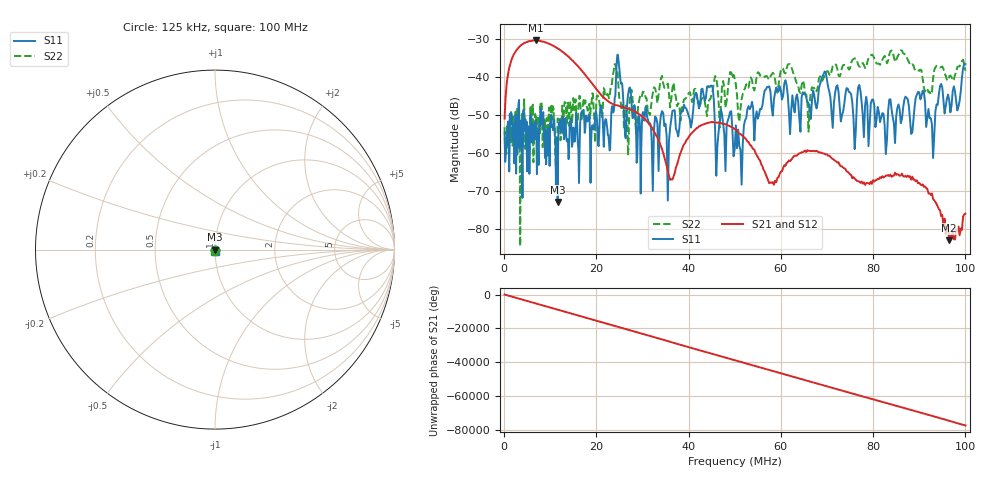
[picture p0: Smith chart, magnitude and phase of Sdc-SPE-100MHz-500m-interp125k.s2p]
!Keysight Technologies PLTS 2019, Build 20190114.1
!FILE: C:\Users\fxb06141\Documents\BUREAU - 2022\IEEE802.3\IEEE802.3dg\Cable modeling\125kHz Interpolation\SPE-100MHz-500m-interp125k.s4p
!$DUT_CFG_DESC: Default 4-Port Configuration
!$NUMBER_PORTS: 4
!$DIFF_PORT_MAP: 1|2P|2|2P|0|UC|0|UC|
!$PORT_MAP: 1|1|<<<<<<|2|2|>>>>>>|3|3|<<<<<<|4|4|>>>>>>|
!Date: Tuesday, March 05, 2024, 10:50:46
!S2P File: Measurements: SDC11,SDC12,SDC21,SDC22:
# MHz S  RI  R 50
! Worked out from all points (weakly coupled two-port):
!   800 points, 125 kHz to 100 MHz, reference 50 ohm
!   highest |S21| = -30.26 dB at 6.875 MHz (marker M1); lowest = -83.0 dB at 96.5 MHz (marker M2)
!   lowest |S11| = -72.9 dB at 11.62 MHz (marker M3), VSWR 1.00, Z = 50 + j0.00189 ohm
!   |S11| at or under -10 dB: start of sweep to end of sweep
!   |S22| runs from -84.6 to -32.9 dB; largest |S21 - S12| = 0
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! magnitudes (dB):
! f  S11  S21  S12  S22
! 125 kHz  -54.6  -50.9  -50.9  -53.2
! 2 MHz  -52.3  -34.2  -34.2  -50.3
! 6.875 MHz  -51.3  -30.3  -30.3  -51.8
! 11.62 MHz  -72.9  -32.3  -32.3  -50.8
! 16.88 MHz  -49.1  -38.3  -38.3  -51.3
! 22.75 MHz  -57.1  -46.5  -46.5  -45.6
! 24.75 MHz  -34.8  -47.5  -47.5  -41.3
! 26.5 MHz  -52.4  -48.1  -48.1  -47.5
! 29.25 MHz  -50.0  -49.7  -49.7  -46.4
! 33.5 MHz  -64.7  -56.7  -56.7  -44.6
! 36.38 MHz  -49.9  -67.0  -67.0  -44.2
! 44.62 MHz  -42.4  -51.9  -51.9  -45.8
! 46.12 MHz  -62.0  -51.9  -51.9  -41.3
! 50.12 MHz  -55.8  -53.7  -53.7  -41.1
! 58 MHz  -47.9  -67.8  -67.8  -39.3
! 66.75 MHz  -46.0  -59.4  -59.4  -42.6
! 69.38 MHz  -38.8  -60.1  -60.1  -39.8
! 75.88 MHz  -55.0  -66.5  -66.5  -35.1
! 77 MHz  -42.0  -67.6  -67.6  -37.2
! 83.38 MHz  -47.4  -65.9  -65.9  -34.8
! 96.5 MHz  -46.2  -83.0  -83.0  -39.8
! 100 MHz  -36.5  -76.0  -76.0  -38.2
